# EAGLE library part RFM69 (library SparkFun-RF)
Hope RF RFM69CW ISM Transceiver Module The RFM69CW radio module by HopeRF is a compact, powerful radio transceiver module for swapping data packets in the 868 MHz ISM band, using standard and enhanced FSK modulation. The radio is great for sub-compact designs; just 4mm of mounted height from using an SMD precision crystal. Datasheet
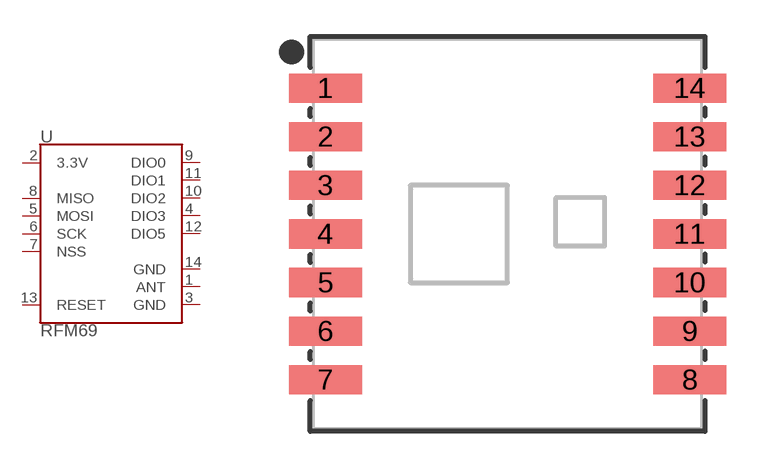
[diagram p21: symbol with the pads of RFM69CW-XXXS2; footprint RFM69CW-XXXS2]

Designator prefix U

## RFM69CW-915MHZ (PROD_ID: IC-11996; VALUE: 915MHz)  [RFM69CW-XXXS2]
1  ANT  pas
2  3.3V  pwr
3  GND  pwr
4  DIO3
5  MOSI  in
6  SCK  in
7  NSS  in
8  MISO
9  DIO0
10  DIO2
11  DIO1
12  DIO5
13  RESET  in
14  GND  pwr

## Footprint RFM69CW-XXXS2 (pad centres in mm)
Hope RF RFM69CW RF Transciever Datasheet
smd 3 x 1.2: 1 -7.5,6; 2 -7.5,4; 3 -7.5,2; 4 -7.5,0; 5 -7.5,-2; 6 -7.5,-4; 7 -7.5,-6; 8 7.5,-6; 9 7.5,-4; 10 7.5,-2; 11 7.5,0; 12 7.5,2; 13 7.5,4; 14 7.5,6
